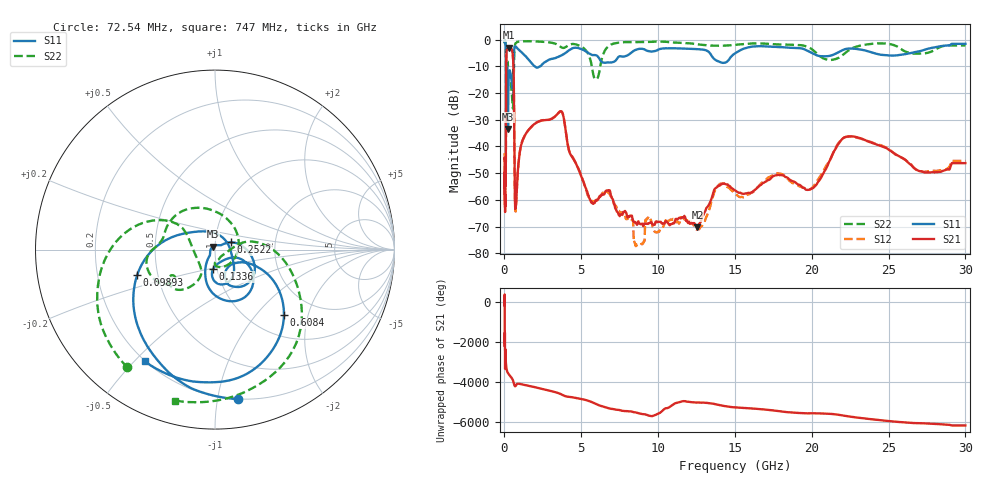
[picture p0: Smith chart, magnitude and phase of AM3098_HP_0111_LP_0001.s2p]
! Date/Time: Thu, Feb 28, 2019 8:38 AM
! Network Analyzer: Agilent Technologies E8364B Rev: A.07.50.67
! Sweep from 0.010 to 30.000 GHz, 1601 Points, Sweep Type: LOG
! Power Supply: 5.022 V, 0.002 A
# Hz S DB R 50
!freq MagS11 AngS11 MagS21 AngS21 MagS12 AngS12 MagS22 AngS22
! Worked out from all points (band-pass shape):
!   1601 points, 10 MHz to 30 GHz, reference 50 ohm
!   highest |S21| = -3.03 dB at 267.8 MHz (marker M1); lowest = -70.2 dB at 12.56 GHz (marker M2)
!   |S21| within 3 dB of the highest: 121 MHz to 546.7 MHz (425.6 MHz wide, 127 % of centre)
!   lowest |S11| = -33.4 dB at 232.8 MHz (marker M3), VSWR 1.04, Z = 48.7 + j1.68 ohm
!   |S11| at or under -10 dB: 102.2 MHz to 571.4 MHz (469.2 MHz wide, 139 % of centre); 1.964 GHz to 2.334 GHz (370.2 MHz wide, 17.2 % of centre)
!   |S22| runs from -25.9 to -0.5 dB; largest |S21 - S12| = 0.012
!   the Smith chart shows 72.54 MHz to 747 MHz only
!   S11 on the Smith chart (normalised r, x): 72.54 MHz: 0.20, -1.15; 98.93 MHz: 0.38, -0.13; 133.6 MHz: 0.96, -0.21; 252.2 MHz: 1.19, +0.10; 608.4 MHz: 1.40, -1.43; 747 MHz: 0.20, -0.54
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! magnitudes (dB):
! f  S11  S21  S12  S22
! 10 MHz  -0.4  -44.5  -43.0  -0.5
! 38.04 MHz  -0.4  -59.4  -57.8  -0.8
! 72.54 MHz  -1.5  -52.5  -53.8  -1.7
! 85.57 MHz  -2.6  -52.4  -52.9  -2.8
! 98.93 MHz  -6.8  -26.1  -26.2  -7.8
! 133.6 MHz  -19.3  -4.7  -4.7  -10.6
! 144.7 MHz  -20.3  -4.1  -4.0  -11.3
! 186.8 MHz  -11.0  -3.6  -3.6  -8.2
! 232.8 MHz  -33.4  -3.2  -3.1  -10.0
! 252.2 MHz  -20.1  -3.1  -3.0  -10.4
! 267.8 MHz  -15.8  -3.0  -3.0  -10.6
! 550.5 MHz  -13.6  -6.3  -6.2  -25.9
! 608.4 MHz  -5.5  -16.7  -16.6  -10.5
! 682.6 MHz  -2.6  -60.2  -59.6  -2.1
! 747 MHz  -2.7  -62.0  -62.7  -1.2
! 2.084 GHz  -10.5  -31.1  -31.1  -0.7
! 3.704 GHz  -6.0  -26.9  -26.9  -2.9
! 5.959 GHz  -5.9  -60.5  -60.2  -15.0
! 7.926 GHz  -6.1  -64.8  -67.2  -1.0
! 12.56 GHz  -3.6  -70.2  -70.8  -1.8
! 22.56 GHz  -3.4  -36.2  -36.3  -3.5
! 30 GHz  -1.6  -46.2  -45.4  -2.2
